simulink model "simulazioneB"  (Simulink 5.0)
settings: Solver=ode45  StartTime=0.0  StopTime=5  RelTol=1e-3
undefined symbols (not defined in the file or in its folder): incrmax, pwm, rpm_to_pwm, sample, sigbuilder_block, TAU
libraries: powerlib_extras x1, fuzblock x1

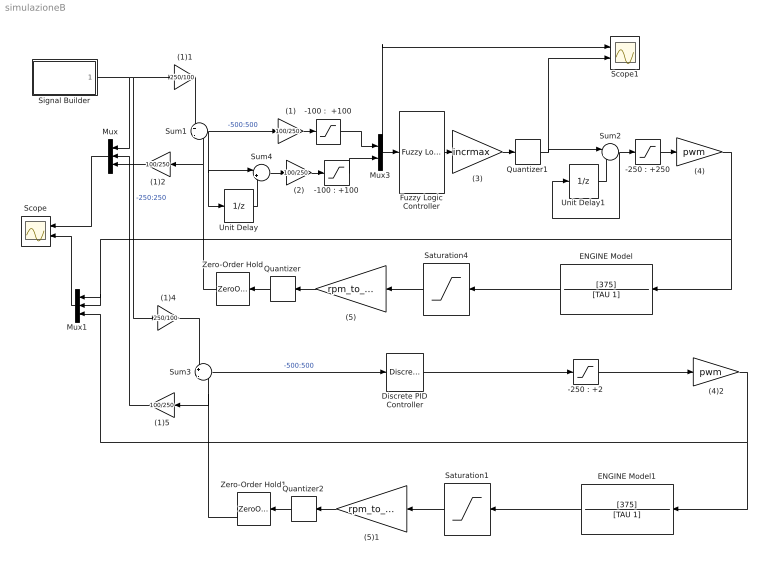
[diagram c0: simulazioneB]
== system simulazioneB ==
  (1) : Gain  Gain=100/250
  (1)1 : Gain  Gain=250/100
  (1)2 : Gain  Orientation=left  Gain=100/250
  (1)4 : Gain  Gain=250/100
  (1)5 : Gain  Orientation=left  Gain=100/250
  (2) : Gain  Gain=100/250
  (3) : Gain  Gain=incrmax
  (4) : Gain  Gain=pwm
  (4)2 : Gain  Gain=pwm
  (5) : Gain  Orientation=left  Gain=rpm_to_pwm
  (5)1 : Gain  Orientation=left  Gain=rpm_to_pwm
  "-100 :  +100" : Saturate  UpperLimit=100  LowerLimit=-100
  "-100 : +100" : Saturate  UpperLimit=100  LowerLimit=-100
  "-250 : +2" : Saturate  UpperLimit=250  LowerLimit=-250
  "-250 : +250" : Saturate  UpperLimit=250  LowerLimit=-250
  Discrete PID Controller : powerlib_extras/Discrete  Control Blocks/Discrete PID Controller  Kp=0.8  Ki=10  Kd=0  TcD=0.0005  Par_Limits=[250 -250]  Init=0  Ts=sample
  ENGINE Model : TransferFcn  Orientation=left  Numerator=[375]  Denominator=[TAU 1]
  ENGINE Model1 : TransferFcn  Orientation=left  Numerator=[375]  Denominator=[TAU 1]
  Fuzzy Logic Controller : fuzblock/Fuzzy Logic  Controller  fis=changeError
  Mux : Mux  Orientation=left  Inputs=3
  Mux1 : Mux  Orientation=left  Inputs=3
  Mux3 : Mux  Inputs=2
  Quantizer : Quantizer  Orientation=left  QuantizationInterval=1
  Quantizer1 : Quantizer  QuantizationInterval=1
  Quantizer2 : Quantizer  Orientation=left  QuantizationInterval=1
  Saturation1 : Saturate  Orientation=left  UpperLimit=6610  LowerLimit=-6610  ZeroCross=off
  Saturation4 : Saturate  Orientation=left  UpperLimit=6610  LowerLimit=-6610  ZeroCross=off
  Scope : Scope  NumInputPorts=2
  Scope1 : Scope  NumInputPorts=2
  Signal Builder : Subsystem  Tag=STV Subsys  LoadFcn=sigbuilder_block('open',[70.5 58.5 519.75 399.75 ]);  StartFcn=sigbuilder_block('start');  StopFcn=sigbuilder_block('stop');  ClipboardFcn=sigbuilder_block('clipboard');
  Sum1 : Sum  Inputs=+|-
  Sum2 : Sum  Inputs=|++
  Sum3 : Sum  Inputs=+|-
  Sum4 : Sum  Inputs=|+-
  Unit Delay : UnitDelay  SampleTime=sample
  Unit Delay1 : UnitDelay  SampleTime=sample
  Zero-Order Hold : ZeroOrderHold  Orientation=left  SampleTime=sample
  Zero-Order Hold1 : ZeroOrderHold  Orientation=left  SampleTime=sample
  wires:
  Mux3/1 -> Fuzzy Logic Controller/1, Scope1/1
  Fuzzy Logic Controller/1 -> (3)/1
  Sum1/1 -> Unit Delay/1, Sum4/1, (1)/1  "-500:500"
  Unit Delay/1 -> Sum4/2
  (4)/1 -> ENGINE Model/1, Mux1/2, Mux1/1
  "-250 : +250"/1 -> (4)/1
  Sum4/1 -> (2)/1
  "-100 : +100"/1 -> Mux3/2
  "-100 :  +100"/1 -> Mux3/1
  (1)/1 -> "-100 :  +100"/1
  (2)/1 -> "-100 : +100"/1
  (5)/1 -> Quantizer/1
  Signal Builder/1(Signal 1) -> Mux/1, (1)1/1, (1)4/1  "-250:250"
  (1)1/1 -> Sum1/1
  ENGINE Model/1 -> Saturation4/1
  Saturation4/1 -> (5)/1
  Mux/1 -> Scope/1
  (1)2/1 -> Mux/2
  (3)/1 -> Quantizer1/1
  Quantizer/1 -> Zero-Order Hold/1
  Unit Delay1/1 -> Sum2/2
  Sum2/1 -> "-250 : +250"/1, Unit Delay1/1
  Quantizer1/1 -> Scope1/2, Sum2/1
  Zero-Order Hold/1 -> Sum1/2, (1)2/1
  (4)2/1 -> ENGINE Model1/1, Mux1/3
  "-250 : +2"/1 -> (4)2/1
  (5)1/1 -> Quantizer2/1
  ENGINE Model1/1 -> Saturation1/1
  Saturation1/1 -> (5)1/1
  Quantizer2/1 -> Zero-Order Hold1/1
  Sum3/1 -> Discrete PID Controller/1  "-500:500"
  (1)4/1 -> Sum3/1
  (1)5/1 -> Mux/3
  Zero-Order Hold1/1 -> (1)5/1, Sum3/2
  Discrete PID Controller/1 -> "-250 : +2"/1
  Mux1/1 -> Scope/2

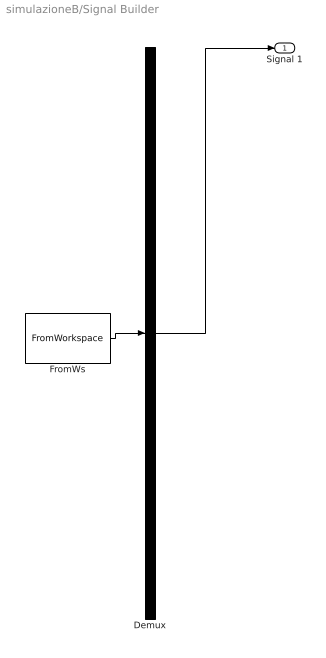
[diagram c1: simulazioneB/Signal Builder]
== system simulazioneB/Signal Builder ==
  Demux : Demux  Tag=STV Demux  Outputs=1
  FromWs : FromWorkspace  Tag=STV FromWs  VariableName=tuvar  SampleTime=0  SigBuilderData=DataTag0
  Signal 1 : Outport  Tag=STV Outport
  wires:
  Demux/1 -> Signal 1/1
  FromWs/1 -> Demux/1
